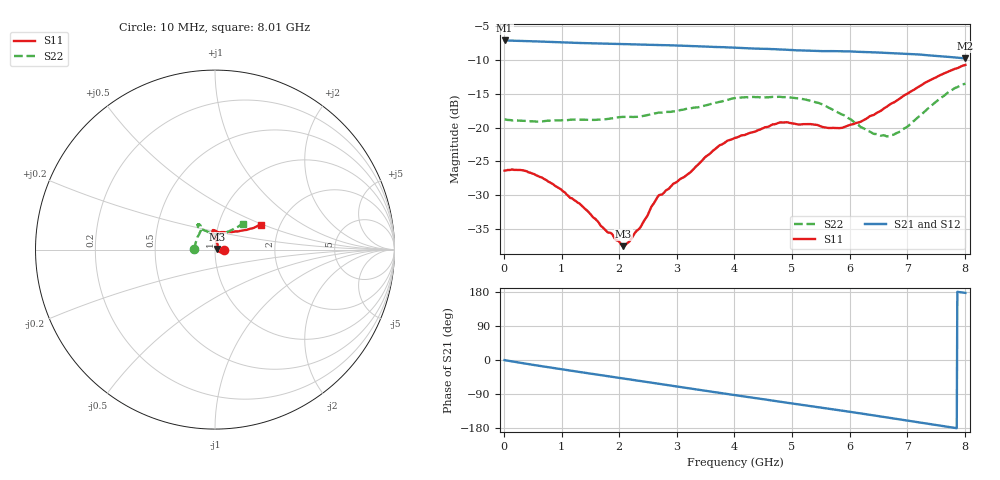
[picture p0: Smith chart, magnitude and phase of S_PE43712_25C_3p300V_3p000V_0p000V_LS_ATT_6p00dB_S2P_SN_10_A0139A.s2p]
! DEVICE ID: PE43712
! File Path: z:\PE43713\PE43713_CHAR_NOM_04292014\AMB\3p300\LS_ATT_6p00dB\PE43713_AMB_3p300V_3p000V_0p000V_LS_ATT_6p00dB_S2P_SN_10_A0139A.s2p
! Serial: 10
! Lot: A0139A
! Temp: 25C
! VDD: 3.300
! VSS: 0.000
! Control_Hi: 3.000
! Control_Lo: 0.000
! Attenuation Step: 6.00dB
! Port 1: RF1
! Port 2: RF2
! ThroughPath:1-2
! IDD: 0.0001470932
! ISS: -8.72e-008
#  Hz  S  RI  R  50
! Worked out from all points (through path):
!   801 points, 10 MHz to 8.01 GHz, reference 50 ohm
!   highest |S21| = -7.12 dB at 10 MHz (marker M1); lowest = -9.8 dB at 8 GHz (marker M2)
!   group delay of S21, straight-line fit = 62.8 ps
!   lowest |S11| = -37.5 dB at 2.07 GHz (marker M3), VSWR 1.03, Z = 51.3 + j0.295 ohm
!   |S11| at or under -10 dB: start of sweep to end of sweep
!   |S22| runs from -21.3 to -13.5 dB; largest |S21 - S12| = 0.0014
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1e7  0.0481 -8.33e-05  0.4407 -0.00255  0.4406 -0.00238  -0.1151 0.000686
3.3e8  0.0475 -0.00906  0.4321 -0.0649  0.4316 -0.0644  -0.1119 0.00977
6.3e8  0.0409 -0.0137  0.4162 -0.1181  0.4162 -0.1181  -0.1095 0.0183
9.6e8  0.0323 -0.0149  0.3915 -0.1714  0.3917 -0.1715  -0.1095 0.0281
1.35e9  0.0233 -0.0124  0.3559 -0.2267  0.3559 -0.2268  -0.1071 0.04
2.07e9  0.013 0.00288  0.273 -0.3117  0.2731 -0.3116  -0.0989 0.0679
2.17e9  0.0132 0.00551  0.2599 -0.3215  0.26 -0.3213  -0.0968 0.0713
2.36e9  0.0129 0.0128  0.2334 -0.3387  0.2334 -0.3385  -0.0906 0.08
2.68e9  0.0151 0.0275  0.1877 -0.3612  0.1877 -0.3613  -0.0815 0.1001
3.23e9  0.00722 0.046  0.1027 -0.3876  0.1028 -0.3877  -0.0782 0.1147
3.72e9  0.00228 0.0726  0.0265 -0.3931  0.0263 -0.393  -0.0801 0.1317
4.01e9  -0.00378 0.0837  -0.0185 -0.3895  -0.0185 -0.3895  -0.0881 0.1398
4.79e9  -0.0123 0.1085  -0.1292 -0.3553  -0.1292 -0.3556  -0.0972 0.1381
5.35e9  -0.000586 0.1057  -0.1965 -0.3133  -0.1964 -0.3131  -0.0938 0.1263
5.63e9  0.0122 0.0986  -0.2265 -0.2896  -0.2264 -0.2898  -0.0787 0.1167
5.87e9  0.0259 0.0961  -0.253 -0.2657  -0.2526 -0.2658  -0.0616 0.1087
6.39e9  0.0735 0.0984  -0.2969 -0.204  -0.2963 -0.2038  -0.0166 0.0897
6.68e9  0.1071 0.0997  -0.315 -0.1652  -0.3147 -0.1651  0.014 0.0854
6.9e9  0.1327 0.1019  -0.3259 -0.1348  -0.3256 -0.1348  0.036 0.0876
7.7e9  0.2254 0.1258  -0.333 -0.0213  -0.3327 -0.0216  0.1281 0.1279
8e9  0.2543 0.1389  -0.3242 0.0156  -0.3237 0.0151  0.1528 0.1443
8.01e9  0.2551 0.1396  -0.3242 0.0166  -0.3235 0.016  0.1534 0.1449
